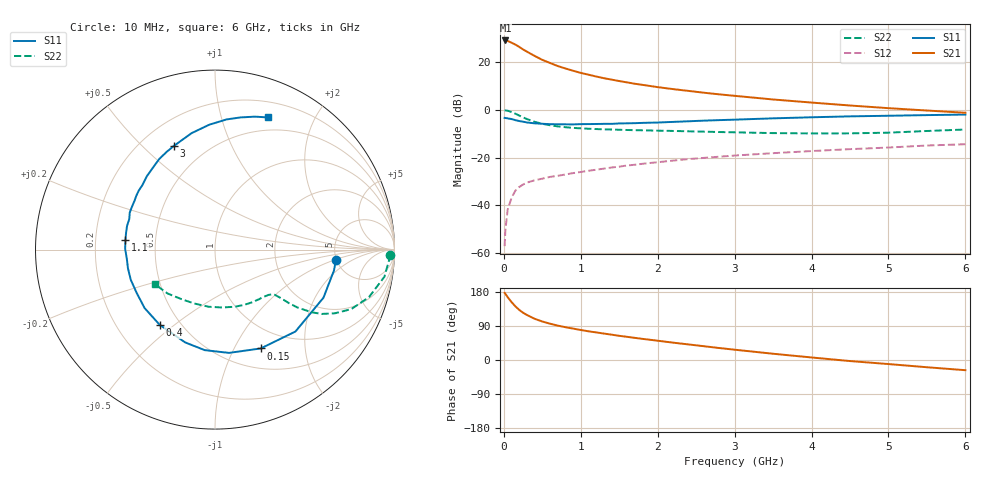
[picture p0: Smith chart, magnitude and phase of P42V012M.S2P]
! SIEMENS Small Signal Semiconductors
! BFP182
! Si NPN RF Bipolar Junction Transistor in SOT143
! VCE = 2 V  IC = 12 mA
! Common Emitter S-Parameters:  March  1996
# GHz  S  MA  R  50
!  f  S11  S21  S12  S22
! GHz  MAG  ANG  MAG  ANG  MAG  ANG  MAG  ANG
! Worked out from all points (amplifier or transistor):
!   36 points, 10 MHz to 6 GHz, reference 50 ohm
!   highest |S21| = 29.0 dB at 20 MHz (marker M1)
!   |S21| within 3 dB of that: start of sweep to 214.4 MHz
!   unconditionally stable (mu >= 1): 981.5 MHz to 5.404 GHz
!   at 250 MHz: K = 0.38, MSG = 28.3 dB, |S12| = -31.3 dB
!   at 1.4 GHz: K = 1.13, MAG = 16.2 dB, |S12| = -24.2 dB
!   at 6 GHz: K = 0.93, MSG = 6.6 dB, |S12| = -14.4 dB
!   S11 on the Smith chart (normalised r, x): 10 MHz: 4.96, -1.01; 150 MHz: 0.74, -1.28; 400 MHz: 0.39, -0.44; 1.1 GHz: 0.33, +0.05; 3 GHz: 0.33, +0.63; 6 GHz: 0.36, +1.42
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0.01  0.6762 -4.7  27.88 177.2  0.0014 84.3  0.9761 -1.7
0.02  0.6731 -9.9  28.22 174.6  0.003 82.5  0.9713 -3.6
0.05  0.6611 -23.9  27.56 165.8  0.0082 81.6  0.956 -9.1
0.1  0.6397 -45.5  25.35 152.9  0.0144 69.0  0.8975 -17.2
0.15  0.6068 -65.2  23.12 141.5  0.0203 61.3  0.8285 -23.6
0.2  0.5807 -82.3  20.69 132.3  0.0242 56.6  0.7561 -28.0
0.25  0.563 -95.9  18.31 124.7  0.0273 53.0  0.694 -31.1
0.3  0.5431 -107.9  16.46 118.8  0.0299 49.9  0.6405 -33.0
0.4  0.5201 -126.4  13.38 108.8  0.0335 47.2  0.5604 -35.1
0.5  0.5099 -140.3  11.08 101.6  0.0362 45.0  0.5087 -35.9
0.6  0.4987 -151.2  9.535 95.8  0.0394 45.3  0.4746 -36.2
0.7  0.4985 -160.4  8.228 90.8  0.0415 45.1  0.4494 -36.5
0.9  0.494 -174.3  6.561 82.9  0.0473 46.6  0.4179 -37.1
1.1  0.502 173.8  5.424 75.7  0.0529 47.0  0.4014 -38.6
1.5  0.5175 156.7  3.993 63.8  0.0646 47.5  0.382 -42.8
1.8  0.5315 145.5  3.324 55.8  0.074 47.2  0.372 -47.1
2.2  0.558 132.9  2.708 45.8  0.0864 45.3  0.3608 -53.8
3  0.6216 111.6  1.959 27.2  0.1102 40.0  0.3376 -70.5
3.5  0.662 101.3  1.643 16.5  0.1236 35.8  0.3251 -82.8
4.5  0.7282 84.9  1.229 -2.8  0.15 28.2  0.3211 -110.2
5.5  0.7734 73.3  0.965 -19.1  0.1787 20.4  0.36 -137.2
6  0.7941 68.0  0.866 -26.9  0.1902 15.5  0.3862 -149.9
